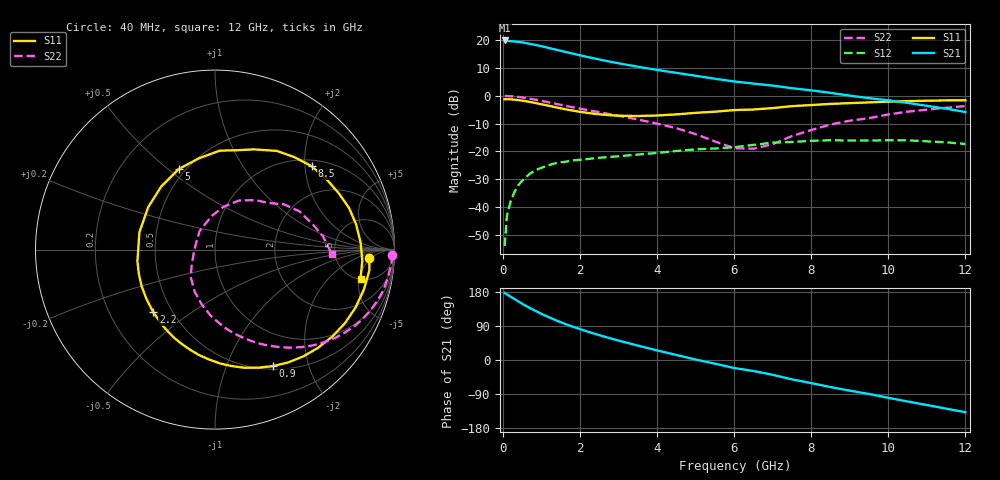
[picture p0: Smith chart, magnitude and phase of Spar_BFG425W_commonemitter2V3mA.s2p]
! Filename: 23bfg425.001
! BFG425W Field C1
! V1=8.180E-001V,V2=2.000E+000V, I1=3.890E-005A, I2=3.000E-003A
# GHz  S  MA  R 50
!  S11  S21  S12  S22
!Freq(GHz)  Mag  Ang  Mag  Ang  Mag  Ang  Mag  Ang
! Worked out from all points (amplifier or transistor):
!   44 points, 40 MHz to 12 GHz, reference 50 ohm
!   highest |S21| = 19.8 dB at 40 MHz (marker M1)
!   |S21| within 3 dB of that: start of sweep to 1.281 GHz
!   unconditionally stable (mu >= 1): 2.838 GHz to end of sweep
!   at 700 MHz: K = 0.23, MSG = 23.3 dB, |S12| = -28.0 dB
!   at 2.4 GHz: K = 0.84, MSG = 17.8 dB, |S12| = -22.4 dB
!   at 12 GHz: K = 1.63, MAG = 1.1 dB, |S12| = -17.3 dB
!   S11 on the Smith chart (normalised r, x): 40 MHz: 12, -4; 900 MHz: 0.54, -1.48; 2.2 GHz: 0.39, -0.36; 5 GHz: 0.46, +0.54; 8.5 GHz: 1.16, +2.17; 12 GHz: 5.05, -5.23
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0.04  0.861 -3.2  9.781 176.8  0.002 79.3  0.987 -1.7
0.1  0.868 -7.5  9.587 173.3  0.007 86.3  0.986 -4.4
0.2  0.859 -14.9  9.487 166.7  0.013 80.2  0.976 -9.0
0.3  0.847 -22.4  9.367 160.8  0.019 75.7  0.966 -13.3
0.5  0.813 -36.7  9.034 148.3  0.03 67.0  0.929 -21.6
0.7  0.772 -50.4  8.489 137.1  0.04 58.8  0.883 -29.3
0.9  0.725 -63.5  7.98 126.6  0.048 51.8  0.832 -36.2
1.2  0.656 -81.7  7.14 112.3  0.057 42.9  0.756 -45.2
1.5  0.594 -98.7  6.376 99.7  0.064 35.7  0.685 -52.9
1.8  0.542 -114.7  5.697 88.3  0.069 30.0  0.622 -59.7
2.2  0.49 -134.5  4.931 74.8  0.073 24.2  0.551 -67.9
2.6  0.457 -153.5  4.311 62.6  0.078 19.6  0.49 -75.6
3  0.437 -171.6  3.809 51.2  0.082 15.8  0.436 -83.2
3.5  0.432 167.2  3.305 37.9  0.088 11.5  0.374 -93.0
4.5  0.462 130.5  2.563 13.3  0.102 2.3  0.261 -115.6
5  0.492 114.4  2.276 1.3  0.109 -4.0  0.204 -131.6
6  0.552 87.2  1.8 -21.1  0.119 -16.1  0.114 178.8
6.5  0.565 78.4  1.647 -29.1  0.131 -16.0  0.112 159.9
7.5  0.649 57.9  1.363 -51.1  0.148 -33.9  0.189 95.3
8.5  0.712 40.6  1.125 -71.5  0.159 -50.0  0.304 64.1
10.5  0.799 10.1  0.743 -109.5  0.158 -84.1  0.517 24.3
12  0.827 -11.4  0.509 -137.8  0.136 -114.6  0.65 -1.9
